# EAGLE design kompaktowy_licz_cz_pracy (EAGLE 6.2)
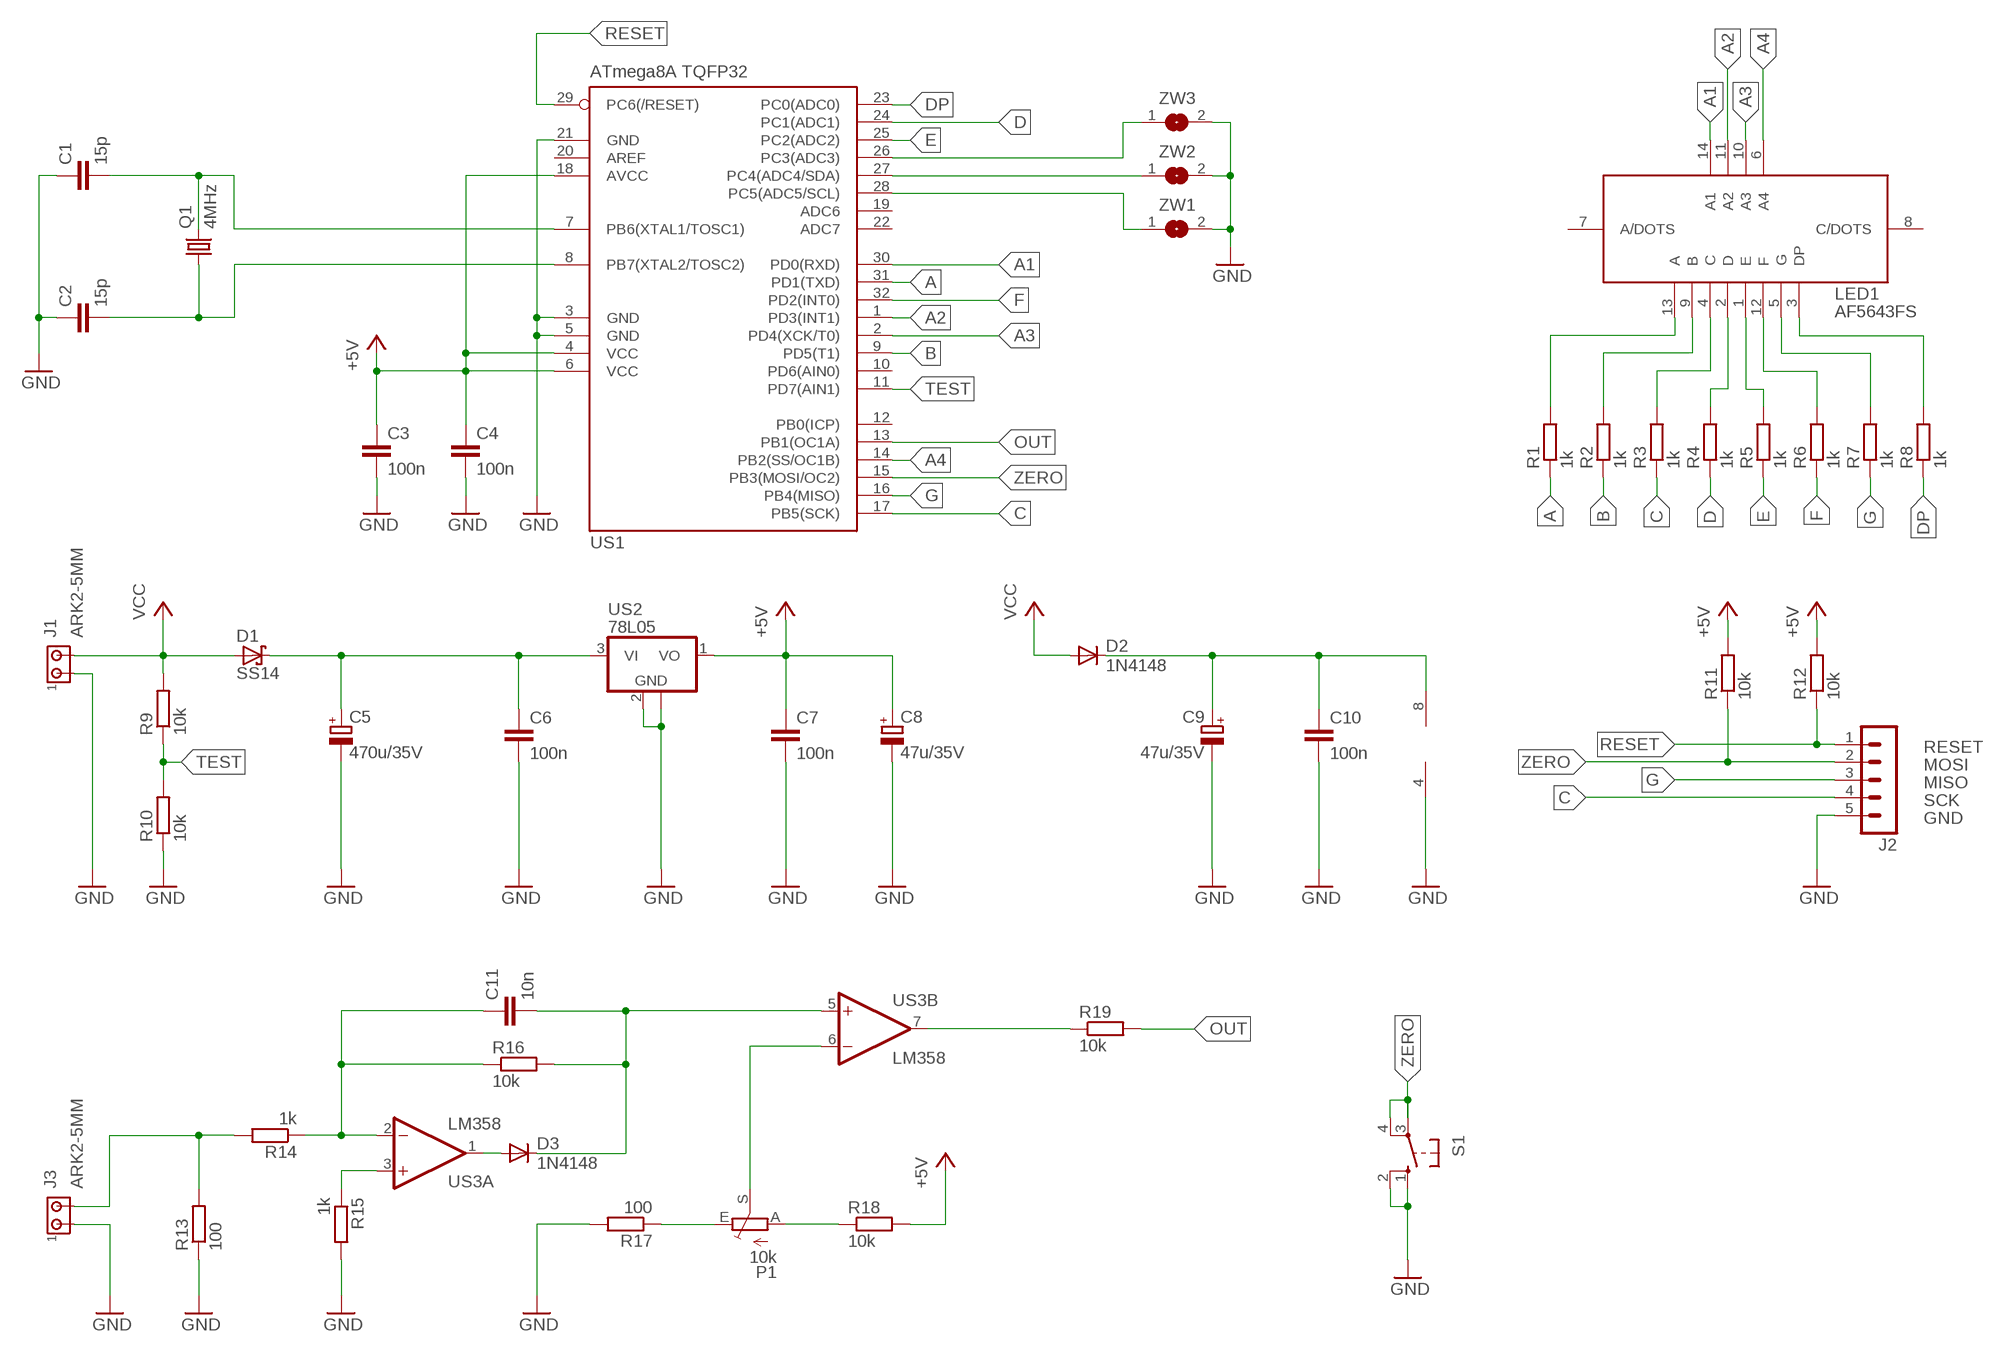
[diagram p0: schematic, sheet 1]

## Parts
C1  15p  C-EUC1206  [C1206]
C2  15p  C-EUC1206  [C1206]
C3  100n  C-EUC1206  [C1206]
C4  100n  C-EUC1206  [C1206]
C5  470u/35V  CPOL-EUE5-10.5  [E5-10,5]
C6  100n  C-EUC1206  [C1206]
C7  100n  C-EUC1206  [C1206]
C8  47u/35V  CPOL-EUE2.5-5  [E2,5-5]
C9  47u/35V  CPOL-EUE2.5-5  [E2,5-5]
C10  100n  C-EUC1206  [C1206]
C11  10n  C-EUC1206  [C1206]
D1  SS14  SCHOTTKY-DIODESMD  [SMB]
D2  1N4148  DIODE-MINIMELF  [MINIMELF]
D3  1N4148  DIODE-MINIMELF  [MINIMELF]
J1  ARK2-5MM  [2PIN-5MM]
J2  MA05-1  [MA05-1]
J3  ARK2-5MM  [2PIN-5MM]
LED1  AF5643FS  LED_DISP_AF5643FS  [LED_DISP_AF5643FS]
P1  10k  TRIM_EU-CA6V  [CA6V]
Q1  4MHz  CRYSTALHC49U-V  [HC49U-V]
R1  1k  R-EU_R1206  [R1206]
R2  1k  R-EU_R1206  [R1206]
R3  1k  R-EU_R1206  [R1206]
R4  1k  R-EU_R1206  [R1206]
R5  1k  R-EU_R1206  [R1206]
R6  1k  R-EU_R1206  [R1206]
R7  1k  R-EU_R1206  [R1206]
R8  1k  R-EU_R1206  [R1206]
R9  10k  R-EU_R1206  [R1206]
R10  10k  R-EU_R1206  [R1206]
R11  10k  R-EU_R1206  [R1206]
R12  10k  R-EU_R1206  [R1206]
R13  100  R-EU_R1206  [R1206]
R14  1k  R-EU_R1206  [R1206]
R15  1k  R-EU_R1206  [R1206]
R16  10k  R-EU_R1206  [R1206]
R17  100  R-EU_R1206  [R1206]
R18  10k  R-EU_R1206  [R1206]
R19  10k  R-EU_R1206  [R1206]
S1  10-XX  [B3F-10XX]
US1  ATmega8A TQFP32  MEGA8-AI  [TQFP32-08]
US2  78L05  78L05F  [SOT89]
US3  LM358  LM358D  [SO08]
ZW1  SJW  [SJW]
ZW2  SJW  [SJW]
ZW3  SJW  [SJW]

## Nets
+5V: C3.1 C4.1 C7.1 C8.+ R11.2 R12.2 R18.2 US1.4(VCC) US1.6(VCC) US1.18(AVCC) US2.1(VO)
A: R1.1 US1.31(PD1(TXD))
A1: LED1.14(A1) US1.30(PD0(RXD))
A2: LED1.11(A2) US1.1(PD3(INT1))
A3: LED1.10(A3) US1.2(PD4(XCK/T0))
A4: LED1.6(A4) US1.14(PB2(SS/OC1B))
B: R2.1 US1.9(PD5(T1))
C: J2.4 R3.1 US1.17(PB5(SCK))
D: R4.1 US1.24(PC1(ADC1))
DP: R8.1 US1.23(PC0(ADC0))
E: R5.1 US1.25(PC2(ADC2))
F: R6.1 US1.32(PD2(INT0))
G: J2.3 R7.1 US1.16(PB4(MISO))
GND: C1.1 C2.1 C3.2 C4.2 C5.- C6.2 C7.2 C8.- C9.- C10.2 J1.P$1 J2.5 J3.P$1 R10.1 R13.1 R15.2 R17.2 S1.1(S) S1.2(S1) US1.3(GND) US1.5(GND) US1.21(GND) US2.2(GND) US2.2@1(GND) US3.4(P:V-) ZW1.2 ZW2.2 ZW3.2
N$1: C2.2 Q1.1 US1.8(PB7(XTAL2/TOSC2))
N$2: C1.2 Q1.2 US1.7(PB6(XTAL1/TOSC1))
N$3: R19.1 US3.7(B:OUT)
N$4: US1.27(PC4(ADC4/SDA)) ZW2.1
N$5: US1.26(PC3(ADC3)) ZW3.1
N$6: US1.28(PC5(ADC5/SCL)) ZW1.1
N$7: LED1.13(A) R1.2
N$8: LED1.9(B) R2.2
N$9: LED1.4(C) R3.2
N$10: LED1.2(D) R4.2
N$11: LED1.1(E) R5.2
N$12: LED1.12(F) R6.2
N$13: LED1.5(G) R7.2
N$14: LED1.3(DP) R8.2
N$15: C9.+ C10.1 D2.C US3.8(P:V+)
N$16: C5.+ C6.1 D1.C US2.3(VI)
N$17: J3.P$2 R13.2 R14.2
N$18: C11.1 R14.1 R16.1 US3.2(A:-IN)
N$19: R15.1 US3.3(A:+IN)
N$20: P1.E R17.1
N$21: P1.S US3.6(B:-IN)
N$22: C11.2 D3.C R16.2 US3.5(B:+IN)
N$23: D3.A US3.1(A:OUT)
N$24: P1.A R18.1
OUT: R19.2 US1.13(PB1(OC1A))
RESET: J2.1 R12.1 US1.29(PC6(/RESET))
TEST: R9.1 R10.2 US1.11(PD7(AIN1))
VCC: D1.A D2.A J1.P$2 R9.2
ZERO: J2.2 R11.1 S1.3(P) S1.4(P1) US1.15(PB3(MOSI/OC2))
Unconnected: LED1.7(A/DOTS) LED1.8(C/DOTS) US1.10(PD6(AIN0)) US1.12(PB0(ICP)) US1.19(ADC6) US1.20(AREF) US1.22(ADC7)

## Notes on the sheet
- RESET
- MOSI
- MISO
- SCK
- GND

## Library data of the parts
C1-C4 C6 C7 C10 C11 = rcl:C-EU: CAPACITOR, European symbol
C5 C8 C9 = rcl:CPOL-EU: POLARIZED CAPACITOR, European symbol
D1 = diode:SCHOTTKY-DIODE: Schottky Diode
D2 D3 = diode:DIODE-: DIODE
J1 J3 = zlacza_futrzak:ARK2: ARK 2
J2 = zlacza_futrzak:MA05-1: PIN HEADER; OC_FARNELL: unknown; OC_NEWARK: unknown
LED1 = inne_futrzak:LED_DISP_AF5643FS
P1 = pot:TRIM_EU-: POTENTIOMETER
Q1 = crystal:CRYSTAL: CRYSTAL; OC_FARNELL: 1666969; OC_NEWARK: unknown
R1-R19 = rcl:R-EU_: RESISTOR, European symbol
S1 = switch-omron:10-XX: OMRON SWITCH; MPN: B3F-1000; OC_FARNELL: 176432; OC_NEWARK: 36M3542
US1 = atmel:MEGA8: MICROCONTROLLER 8 Kbytes FLASH, 1 kbytes SRAM, 512 bytes EEPROM, USART, 6-channel 10 bit ADC, 2-channel 8 bit ADC Pin compatible with Atmega48, ATMega88, ATMega168 Source: avr.lbr; MPN: ATMEGA8-16AU; OC_FARNELL: 9171371; OC_NEWARK: 73M8863
US2 = linear:78L*: POSITOIV-VOLTAGE REGULATORS Output up to 100 mA Source: http://focus.ti.com/lit/ds/symlink/ua78l05.pdf
US3 = linear:LM358: OP AMP also LM158; LM258; LM2904 Source: http://cache.national.com/ds/LM/LM158.pdf
ZW1-ZW3 = jumper:SJ: SMD solder JUMPER

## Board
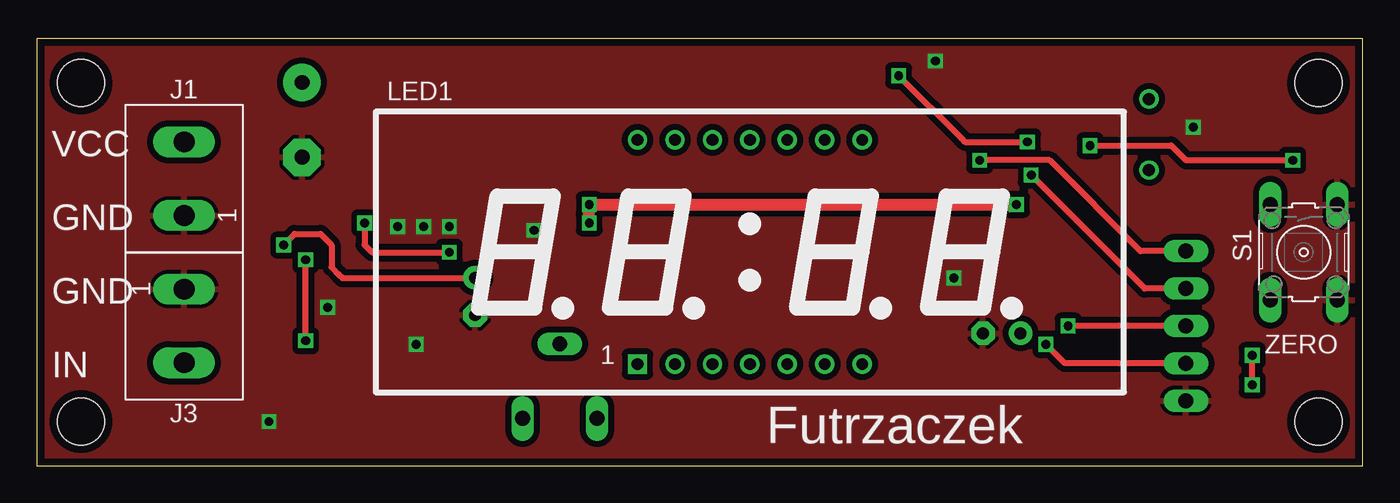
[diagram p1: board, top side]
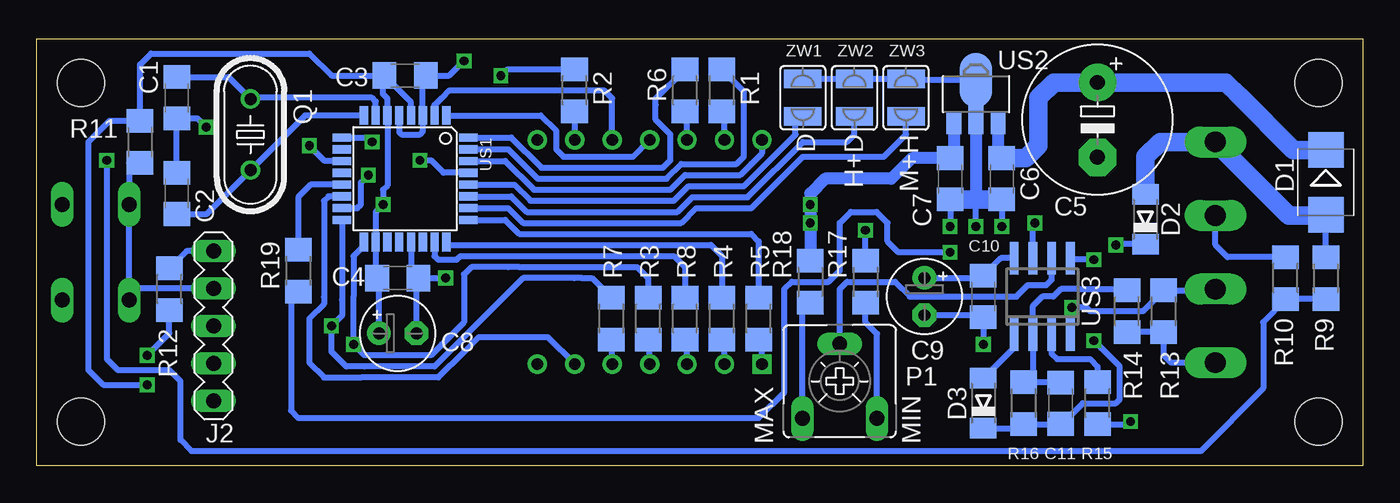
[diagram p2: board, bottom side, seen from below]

Size 90 x 29 mm. Coordinates in mm from the lower left corner, seen from the top.
Outline: 0,0 90,0 90,29 0,29 0,0
Copper layers (1*16): Top 0.035mm / dielectric 1.5mm / Bottom 0.035mm
Design rules: minimum track width 10mil, minimum drill 23mil, track to track 8mil, track to pad 8mil, pad to pad 8mil, via to via 8mil, smd to smd 8mil, copper to edge 20mil, drill to drill 8mil, minimum pad ring 10mil, minimum via ring 8mil, stop-mask expansion 4mil, vias tented up to drill 0mil, thermal gap 10mil
Holes 3.2 mm at 87,3 87,26 3,3 3,26

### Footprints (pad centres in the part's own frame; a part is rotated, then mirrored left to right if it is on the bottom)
C1206 = smd 1.6 x 1.8: 1 -1.4,0; 2 1.4,0
E5-10,5 = drill 1.016 pad 2.54: + -2.54,0 | drill 1.016 pad 2.54 octagon: - 2.54,0
E2,5-5 = drill 0.813 pad 1.6: + -1.27,0 | drill 0.813 pad 1.6 octagon: - 1.27,0
SMB = smd 2.4 x 2.4: A 2.2,0; C -2.2,0
MINIMELF = smd 1.4 x 1.8: A 1.7,0; C -1.7,0
2PIN-5MM = drill 1.4 long: P$1 -2.5,0; P$2 2.5,0
MA05-1 = drill 1.016 long: 1 -5.08,0; 2 -2.54,0; 3 0,0; 4 2.54,0; 5 5.08,0
LED_DISP_AF5643FS = drill 0.8 square: 1 17.78,1.905 | drill 0.8: 2 20.32,1.905; 3 22.86,1.905; 4 25.4,1.905; 5 27.94,1.905; 6 30.48,1.905; 7 33.02,1.905; 8 33.02,17.145; 9 30.48,17.145; 10 27.94,17.145; 11 25.4,17.145; 12 22.86,17.145; 13 20.32,17.145; 14 17.78,17.145
CA6V = drill 1.016 long: A -2.54,-2.54; E 2.54,-2.54; S 0,2.54
HC49U-V = drill 0.813: 1 -2.413,0; 2 2.413,0
R1206 = smd 1.6 x 1.803: 1 -1.422,0; 2 1.422,0
B3F-10XX = drill 1.016 long: 1 -3.251,2.261; 2 3.251,2.261; 3 -3.251,-2.261; 4 3.251,-2.261
TQFP32-08 = smd 1.27 x 0.559: 1 -4.293,2.8; 2 -4.293,2; 3 -4.293,1.2; 4 -4.293,0.4; 5 -4.293,-0.4; 6 -4.293,-1.2; 7 -4.293,-2; 8 -4.293,-2.8; 17 4.293,-2.8; 18 4.293,-2; 19 4.293,-1.2; 20 4.293,-0.4; 21 4.293,0.4; 22 4.293,1.2; 23 4.293,2; 24 4.293,2.8 | smd 0.559 x 1.27: 9 -2.8,-4.293; 10 -2,-4.293; 11 -1.2,-4.293; 12 -0.4,-4.293; 13 0.4,-4.293; 14 1.2,-4.293; 15 2,-4.293; 16 2.8,-4.293; 25 2.8,4.293; 26 2,4.293; 27 1.2,4.293; 28 0.4,4.293; 29 -0.4,4.293; 30 -1.2,4.293; 31 -2,4.293; 32 -2.8,4.293
SOT89 = smd 1 x 1.5: 1 -1.499,-1.981; 3 1.499,-1.981 | smd 1 x 2: 2 0,-1.727 | smd 2.2 x 3.7: 2@1 0,0.94
SO08 = smd 0.6 x 2.2: 1 -1.905,-2.6; 2 -0.635,-2.6; 3 0.635,-2.6; 4 1.905,-2.6; 5 1.905,2.6; 6 0.635,2.6; 7 -0.635,2.6; 8 -1.905,2.6
SJW = smd 1.27 x 2.54: 1 -1.27,0; 2 1.27,0

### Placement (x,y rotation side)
C1  80.5,25 90 bottom
C2  80.5,18.5 270 bottom
C3  65,26.5 0 bottom
C4  65.5,12.75 0 bottom
C5  18,23.5 270 bottom
C6  24.5,19.5 270 bottom
C7  28,19.5 270 bottom
C8  65.5,9 0 bottom
C9  29.75,11.5 270 bottom
C10  25.75,11.5 270 bottom
C11  20.5,4.25 270 bottom
D1  2.5,19.25 270 bottom
D2  14.75,16.75 90 bottom
D3  25.75,4.25 90 bottom
J1  10,19.5 90 top
J2  78,9.5 270 bottom
J3  10,9.5 270 top
LED1  23,5 0 top
P1  35.5,5.75 0 bottom
Q1  75.5,22.5 90 bottom
R1  43.5,25.5 270 bottom
R2  53.5,25.5 270 bottom
R3  48.5,10 270 bottom
R4  43.5,10 270 bottom
R5  41,10 270 bottom
R6  46,25.5 270 bottom
R7  51,10 270 bottom
R8  46,10 270 bottom
R9  2.5,12.75 90 bottom
R10  5.25,12.75 270 bottom
R11  83,22 90 bottom
R12  81,12 270 bottom
R13  13.5,10.5 270 bottom
R14  16,10.5 270 bottom
R15  18,4.25 270 bottom
R16  23,4.25 270 bottom
R17  33.75,12.5 90 bottom
R18  37.5,12.5 90 bottom
R19  72.25,13.25 90 bottom
S1  86,14.5 270 top
US1  65,19.5 270 bottom
US2  26.25,25.25 0 bottom
US3  21.75,11.5 0 bottom
ZW1  38,25 90 bottom
ZW2  34.5,25 90 bottom
ZW3  31,25 90 bottom

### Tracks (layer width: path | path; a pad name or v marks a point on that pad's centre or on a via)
+5V  (via drill 0.6)
  Top 0.406: v82.5,5.5 v82.5,7.5
  Top 0.813: v66.5,17.75 v37.5,17.75 v37.5,16.5
  Bottom 0.406: C8.+ 66.77,12.62 C4.1 67,12.85 US1.18 67,17.25 v66.5,17.75 66.5,18.75 66.2,19.05 US1.6 66.2,24.95 66.5,25.25 66.5,26.4 C3.1 | US1.4 64.6,24.7 C3.1 | C3.1 70,26.5 71.5,28 82.25,28 83,27.25 R11.2 85.08,23.42 86.5,22 86.5,6.5 85.5,5.5 v82.5,5.5 | v82.5,7.5 81,9 R12.2
  Bottom 0.813: US2.1 27.75,21.15 C7.1 30.6,20.9 32,19.5 36.5,19.5 37.5,18.5 v37.5,17.75 R18.2
A
  Bottom 0.406: US1.31 58,21.5 56,19.5 47.25,19.5 46.25,20.5 42.5,20.5 42,21 42,25.42 R1.1
A1
  Bottom 0.406: US1.30 58.2,20.7 56.25,18.75 47,18.75 46,19.75 42.25,19.75 41.5,20.5 40.78,21.22 LED1.14
A2
  Bottom 0.406: US1.1 55.79,23.79 54.75,22.75 54.75,21.5 54.25,21 49.55,21 LED1.11
A3
  Bottom 0.406: US1.2 63,24.5 62.5,25 62,25.5 51.5,25.5 51,25 50.94,24.94 LED1.10
A4
  Bottom 0.406: US1.14 70.2,18.3 70.5,18 70.5,11.5 70.5,11 71.5,10 71.5,7 70.5,6 68,6 62.75,6 61,7.75 60,8.75 55.33,8.75 LED1.6
B  (via drill 0.6)
  Top 0.406: v58.5,26.5 62.75,22.25 63,22 v67.25,22
  Bottom 0.406: R2.1 58.08,26.92 v58.5,26.5 | 67.5,22.25 v67.25,22 67.55,22.3 US1.9
C  (via drill 0.6)
  Top 0.406: J2.4 69.79,6.96 v68.5,8.25
  Bottom 0.406: US1.17 67.8,14.95 68.5,14.25 68.5,11.5 v68.5,8.25 67.75,7.5 67.5,7.5 63.25,7.5 62.5,8.25 61,9.75 61,13 60.5,13.5 58,13.5 57.25,13.5 49.25,13.5 48.5,12.75 R3.1
D
  Bottom 0.406: US1.24 62.2,15.05 62.25,15 44.25,15 43.5,14.25 R4.1
DP
  Bottom 0.406: US1.23 63,14.25 62.75,14 61.5,14 61.25,14.25 46.75,14.25 46,13.5 R8.1
E
  Bottom 0.406: US1.25 58.2,16.7 57.25,15.75 41.5,15.75 41,15.25 R5.1
F
  Bottom 0.406: US1.32 57.8,22.3 55.75,20.25 47.5,20.25 47,20.75 47,22.5 48,23.5 48,24.5 48,24.92 R6.1 46.08,27
G  (via drill 0.6)
  Top 0.406: J2.3 v70,9.5
  Bottom 0.406: US1.16 69.29,11.29 69.25,11.25 69.25,10.25 v70,9.5 70,7.75 69,6.75 67.75,6.75 63,6.75 61.75,8 57,12.75 53.5,12.75 53,12.75 52.33,12.75 R7.1
GND  (via drill 0.6)
  Bottom 0.406: C8.- 64.23,12.62 C4.2 | US1.21 64.6,13.25 C4.2 | J3.P$1 10.08,11.92 R13.1 14.92,10.5 18.5,10.5 18.75,10.75 v19.75,10.75 19.84,10.65 US3.4 | C9.- 25.88,10.23 C10.2 v25.75,8.25 | C6.2 v24.5,16.25 | v26.25,16.25 26.25,18.25 28,18.25 v28,16.25 | R17.2 v33.75,16 | R15.2 15.92,2.83 v15.75,3 | US1.5 65.4,22.65 65.25,22.5 64,22.5 63.8,22.7 US1.3 63.8,26.3 C3.2 62,26.5 v61,27.5 | C4.2 v62.25,12.75 | US2.2@1 30.92,26.19 ZW3.2 ZW2.2 ZW1.2 | R10.1 9.17,14.17 10,15 J1.P$1 | v78.5,23 79.1,23.6 C1.1 C2.1
  Bottom 0.813: 26.25,18.1 26.25,18.25 US2.2 US2.2@1
  Bottom 1.27: C7.2 26.25,18.1 C6.2
  pour Top (isolate 0.406): 0,0 90,0 90,29 0,29
N$1
  Bottom 0.406: US1.8 71.79,23.79 Q1.1 78.49,17.1 C2.2
N$2
  Bottom 0.406: US1.7 67,24.75 67.25,25 75.41,25 Q1.2 76.99,26.4 C1.2
N$3  (via drill 0.6)
  Top 0.406: v22.25,16.5 22.25,15 22.75,14.5 v28,14.5
  Bottom 0.406: US3.7 22.39,16.36 v22.25,16.5 | R19.1 72.25,11.75 72.75,11.25 72.75,3.75 72.25,3.25 41,3.25 39.25,5 39.25,12 38.75,12.5 36.25,12.5 35.5,13.25 35.5,16.5 34.75,17.25 33,17.25 32.25,16.5 32.25,15.25 31.5,14.5 v28,14.5
N$4
  Bottom 0.406: US1.27 57.8,18.3 56.75,17.25 46.5,17.25 45.5,18.25 41.75,18.25 38,22 35,22 34.5,22.5 ZW2.1
N$5
  Bottom 0.406: US1.26 58,17.5 57,16.5 46.25,16.5 45.25,17.5 41.5,17.5 38,21 32.5,21 31,22.5 ZW3.1
N$6
  Bottom 0.406: US1.28 57.6,19.1 56.5,18 46.75,18 45.75,19 42,19 38.5,22.5 38.5,23.23 ZW1.1
N$7
  Bottom 0.406: LED1.13 43.32,23.9 R1.2
N$8
  Bottom 0.406: LED1.9 53.48,24.06 R2.2
N$9
  Bottom 0.406: LED1.4 48.4,8.48 R3.2
N$10
  Bottom 0.406: LED1.2 43.32,8.4 R4.2
N$11
  Bottom 0.406: LED1.1 40.78,8.36 R5.2
N$12
  Bottom 0.406: LED1.12 45.86,23.94 R6.2
N$13
  Bottom 0.406: LED1.5 50.94,8.52 R7.2
N$14
  Bottom 0.406: LED1.3 45.86,8.44 R8.2
N$15  (via drill 0.6)
  Top 0.406: v16.75,15 17.5,15.75 19.25,15.75 20,15 20,13.5 20.5,13 20.75,12.75 29.73,12.75 C9.+
  Bottom 0.406: US3.8 24.55,14.1 C10.1 25.88,12.77 C9.+ | D2.C 16.7,15.05 v16.75,15
N$16
  Bottom 0.813: US2.3 24.75,21.15 C6.1
  Bottom 1.27: D1.C 4.7,21.45 8.38,25.12 | 8.38,25.12 8.5,25.25 | 8.38,25.12 9.29,26.04 C5.+ 20.96,26.04 22,25 22,21.75 22.75,21 22.85,20.9 C6.1
N$17
  Bottom 0.406: J3.P$2 13,7 13.5,7.5 R13.2 R14.2
N$18
  Bottom 0.406: C11.1 22.98,5.65 R16.1 22.39,6.04 US3.2 22.39,10.87 21.75,11.5 21,11.5 20.5,12 19.25,12 16.33,12 R14.1
N$19
  Bottom 0.406: US3.3 21.11,7.62 20.75,7.25 18.5,7.25 18,6.75 R15.1
N$20
  Bottom 0.406: P1.E 32.96,8.96 33.75,9.75 R17.1
N$21
  Bottom 0.406: P1.S 35.5,12 35,12.5 31.75,12.5 30.75,11.5 23.5,11.5 22.75,12.25 21.5,12.25 21.11,12.63 US3.6
N$22  (via drill 0.6)
  Top 0.406: v18.25,8.5 v18.25,14
  Bottom 0.406: D3.C 23.28,2.55 R16.2 20.52,2.83 C11.2 20.4,2.85 19,4.25 16.75,4.25 16.5,4.5 16.5,6.75 17.75,8 v18.25,8.5 | v18.25,14 19.75,14 US3.5
N$23
  Bottom 0.406: US3.1 23.66,8.04 D3.A
N$24
  Bottom 0.406: P1.A 38.04,11.04 R18.1
OUT
  Bottom 0.406: US1.13 71.4,19.1 72.25,18.25 R19.2
RESET  (via drill 0.6)
  Top 0.406: J2.1 74.92,14.58 68.75,20.75 v64,20.75
  Bottom 0.406: v64,20.75 63.25,20.75 62.4,19.9 US1.29 | J2.1 79.84,14.58 R12.1
TEST  (via drill 0.6)
  Top 0.406: v71.5,21.75 77,21.75 78,20.75 v85.25,20.75
  Bottom 0.406: R9.1 R10.2 5.25,11.25 6.75,9.75 6.75,5.25 11,1 79.5,1 80.25,1.75 80.25,5.75 81,6.5 84.5,6.5 85.25,7.25 v85.25,20.75 | US1.11 70.45,20.7 v71.5,21.75
VCC
  Bottom 0.406: R9.2 D1.A
  Bottom 1.27: D1.A 2.55,17 5,17 J1.P$2 13.75,22 14.75,21 D2.A
ZERO  (via drill 0.6)
  Top 0.406: v67.5,19.75 75.21,12.04 J2.2
  Bottom 0.406: R11.1 83.49,20.57 83.74,20.57 S1.3 83.74,12.04 | J2.2 83.74,12.04 | S1.4 83.74,12.04 | US1.15 68.25,17.5 68,17.75 68,19.25 v67.5,19.75

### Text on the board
tPlace: VCC | GND | GND | ZERO | IN | Futrzaczek
bPlace: H+D | D | M+H | MIN | MAX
